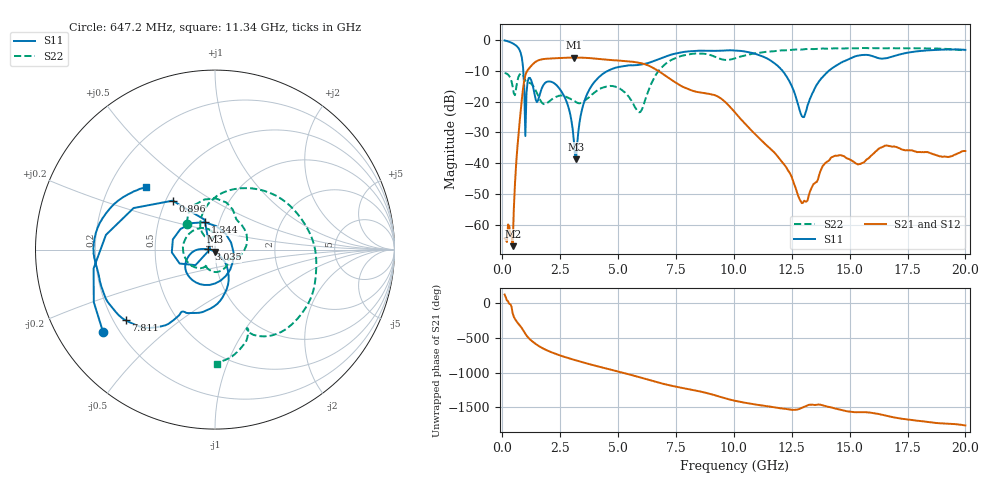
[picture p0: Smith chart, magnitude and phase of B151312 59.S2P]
!  2-Port S-parameters saved by WinCal
! VAR MeasName=S-Parameters (CALIBRATED_DATA) read from VNA (N5244A)
! VAR MeasDate=12/8/2015 5:48:24 PM
! VAR NAME=B151312 59
! VAR FILENAME=B151312 59.S2P
! VAR DATE=12/8/2015 5:48:24 PM
! VAR PHYS_PORTS=1,2
# Hz S DB R 50
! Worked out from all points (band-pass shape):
!   401 points, 100 MHz to 20 GHz, reference 50 ohm
!   highest |S21| = -5.74 dB at 3.085 GHz (marker M1); lowest = -66.9 dB at 448.2 MHz (marker M2)
!   |S21| within 3 dB of the highest: 1.214 GHz to 6.423 GHz (5.209 GHz wide, 136 % of centre)
!   lowest |S11| = -38.7 dB at 3.184 GHz (marker M3), VSWR 1.02, Z = 49.8 - j1.15 ohm
!   |S11| at or under -10 dB: 905.1 MHz to 4.571 GHz (3.666 GHz wide, 134 % of centre); 12.1 GHz to 14.11 GHz (2.007 GHz wide, 15.3 % of centre)
!   |S22| runs from -23.5 to -2.6 dB; largest |S21 - S12| = 0.0019
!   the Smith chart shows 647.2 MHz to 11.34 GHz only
!   S11 on the Smith chart (normalised r, x): 647.2 MHz: 0.14, -0.32; 896 MHz: 0.54, +0.34; 1.344 GHz: 0.85, +0.27; 3.035 GHz: 0.93, +0.00; 7.811 GHz: 0.25, -0.33; 11.34 GHz: 0.36, +0.34
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1e8  -0.20 -22.6  -64.37 122.3  -64.52 117.7  -10.73 165.9
4.4825e8  -1.13 -97.9  -66.90 -146.3  -65.22 -147.7  -15.11 112.9
6.4725e8  -2.21 -143.5  -35.31 82.8  -35.30 82.9  -13.42 137.5
8.96e8  -8.86 130.9  -15.79 -26.7  -15.79 -26.8  -11.38 76.4
1.34375e9  -15.79 110.4  -7.70 156.2  -7.71 156.2  -15.06 7.6
1.692e9  -15.99 -67.8  -6.34 79.3  -6.34 79.3  -20.22 -31.4
2.13975e9  -13.67 -136.9  -6.02 10.2  -6.02 10.2  -19.27 -51.0
3.03525e9  -28.69 178.2  -5.74 -89.9  -5.75 -89.8  -19.44 -117.5
3.085e9  -32.25 -176.7  -5.74 -94.8  -5.74 -94.8  -19.70 -118.0
3.1845e9  -38.70 -97.2  -5.74 -104.5  -5.74 -104.5  -20.19 -119.1
3.43325e9  -22.91 -50.8  -5.79 -128.3  -5.78 -128.3  -20.35 -120.2
5.02525e9  -8.80 -104.1  -6.71 93.4  -6.71 93.4  -15.63 144.7
5.92075e9  -8.10 -118.2  -7.46 13.9  -7.43 13.8  -23.50 109.6
6.7665e9  -6.21 -122.1  -10.22 -65.8  -10.21 -65.9  -9.92 82.4
7.81125e9  -3.95 -141.6  -15.29 -143.3  -15.25 -143.7  -5.07 -0.1
1.005e10  -3.42 174.6  -23.54 34.6  -23.53 34.2  -5.99 -68.5
1.13435e10  -5.68 137.9  -33.72 -39.0  -33.76 -39.3  -3.92 -89.0
1.29355e10  -24.74 14.4  -52.95 -65.0  -52.81 -65.0  -3.14 -112.7
1.338325e10  -17.45 -78.4  -47.63 -21.0  -47.61 -20.9  -2.99 -117.5
1.427875e10  -9.04 -112.5  -37.90 -67.9  -37.90 -67.7  -2.76 -128.9
1.67165e10  -5.73 -156.0  -34.46 168.2  -34.39 168.0  -2.69 -151.7
2e10  -3.24 162.1  -36.05 40.1  -36.16 39.3  -3.40 179.4
